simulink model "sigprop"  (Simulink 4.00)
settings: Solver=ode45  StartTime=0.0  StopTime=10.0  RelTol=1e-3

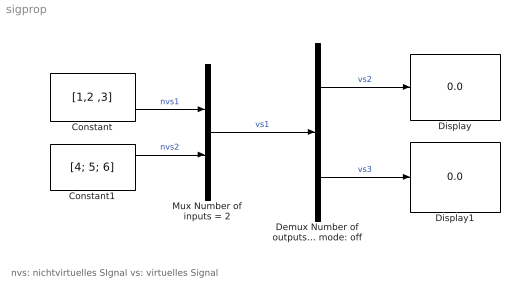
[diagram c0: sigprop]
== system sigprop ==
  note: nvs: nichtvirtuelles SIgnal vs: virtuelles Signal
  Constant : Constant  Value=[1,2 ,3]
  Constant1 : Constant  Value=[4; 5; 6]
  Demux Number of outputs = 2 Bus selection mode: off : Demux  Outputs=2  BusSelectionMode=on
  Display : Display
  Display1 : Display
  Mux Number of inputs = 2 : Mux  Inputs=2
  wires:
  Constant1/1 -> Mux Number of inputs = 2/2  "nvs2"
  Constant/1 -> Mux Number of inputs = 2/1  "nvs1"
  Mux Number of inputs = 2/1 -> Demux Number of outputs = 2 Bus selection mode: off/1  "vs1"
  Demux Number of outputs = 2 Bus selection mode: off/1 -> Display/1  "vs2"
  Demux Number of outputs = 2 Bus selection mode: off/2 -> Display1/1  "vs3"
